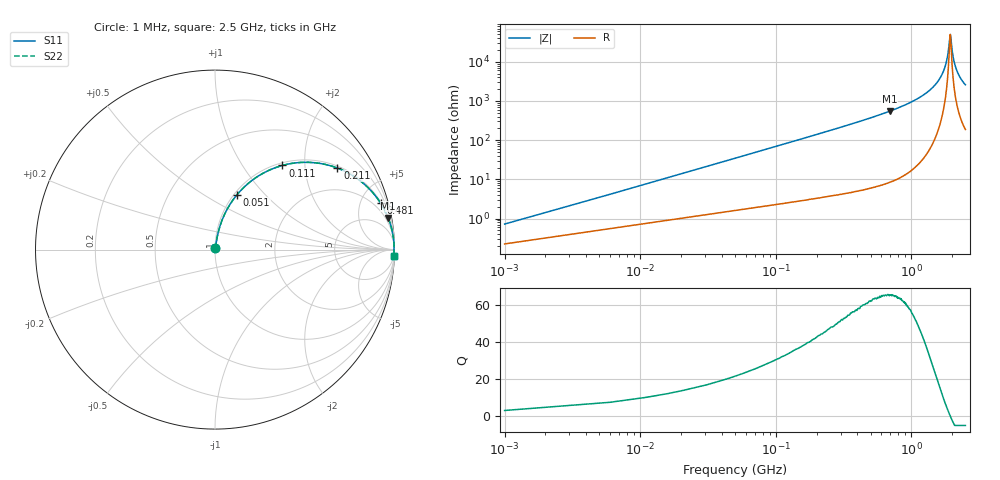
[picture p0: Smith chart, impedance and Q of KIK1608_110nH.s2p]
!version-2
!date-01.2022
!Series
# MHz S RI R 50
!Freq ReS11 ImS11 ReS21 ImS21 ReS12 ImS12 ReS22 ImS22
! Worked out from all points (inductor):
!   501 points, 1 MHz to 2.5 GHz, reference 50 ohm
!   read as one part in series: L = 110 nH near 11 MHz
!   highest Q = 65.2 at 691 MHz (marker M1), where L = 126 nH
!   self-resonance near 1.93 GHz
!   S11 on the Smith chart (normalised r, x): 1 MHz: 1.00, +0.01; 51 MHz: 1.03, +0.71; 111 MHz: 1.05, +1.54; 211 MHz: 1.07, +2.95; 481 MHz: 1.12, +7.09; 2.5 GHz: 5, -51
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1  0.00232 0.00688  0.9977 -0.00688  0.9977 -0.00688  0.00232 0.00688
16  0.0208 0.1073  0.9792 -0.1073  0.9792 -0.1073  0.0208 0.1073
21  0.0303 0.1393  0.9697 -0.1393  0.9697 -0.1393  0.0303 0.1393
36  0.0696 0.2285  0.9304 -0.2285  0.9304 -0.2285  0.0696 0.2285
51  0.1218 0.3048  0.8782 -0.3048  0.8782 -0.3048  0.1218 0.3048
111  0.376 0.469  0.624 -0.469  0.624 -0.469  0.376 0.469
211  0.6816 0.4545  0.3184 -0.4545  0.3184 -0.4545  0.6816 0.4545
421  0.8992 0.2927  0.1008 -0.2927  0.1008 -0.2927  0.8992 0.2927
481  0.9226 0.2591  0.0774 -0.2591  0.0774 -0.2591  0.9226 0.2591
691  0.9652 0.1758  0.0348 -0.1758  0.0348 -0.1758  0.9652 0.1758
836  0.9785 0.1374  0.0215 -0.1374  0.0215 -0.1374  0.9785 0.1374
1255  0.9939 0.0661  0.00608 -0.0661  0.00608 -0.0661  0.9939 0.0661
1500  0.9968 0.0382  0.00316 -0.0382  0.00316 -0.0382  0.9968 0.0382
1670  0.9977 0.0219  0.00227 -0.0219  0.00227 -0.0219  0.9977 0.0219
1825  0.998 0.00866  0.00198 -0.00866  0.00198 -0.00866  0.998 0.00866
1865  0.998 0.00543  0.00197 -0.00543  0.00197 -0.00543  0.998 0.00543
1920  0.998 0.00111  0.002 -0.00111  0.002 -0.00111  0.998 0.00111
1935  0.998 -5.09e-05  0.00202 5.09e-05  0.00202 5.09e-05  0.998 -5.09e-05
2010  0.9979 -0.00571  0.00213 0.00571  0.00213 0.00571  0.9979 -0.00571
2085  0.9977 -0.0112  0.00232 0.0112  0.00232 0.0112  0.9977 -0.0112
2250  0.9971 -0.0225  0.00292 0.0225  0.00292 0.0225  0.9971 -0.0225
2500  0.9957 -0.0384  0.00429 0.0384  0.00429 0.0384  0.9957 -0.0384
